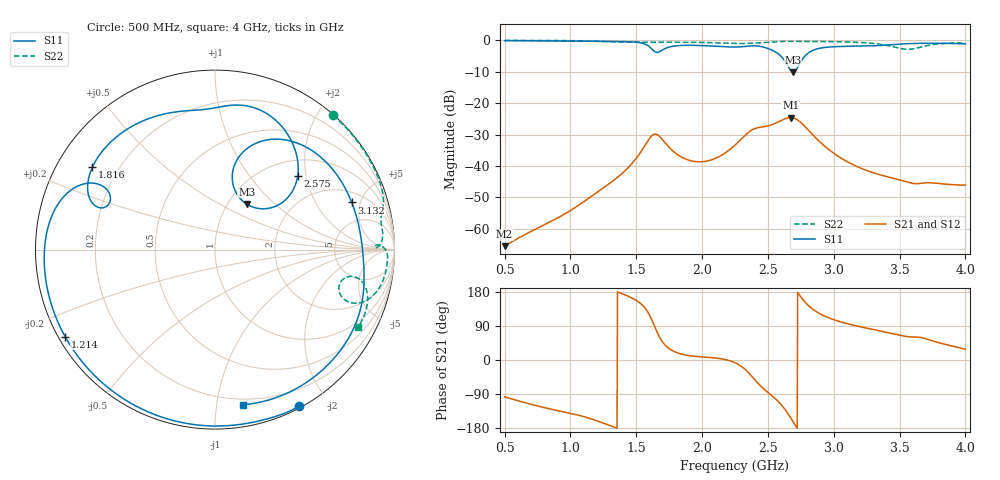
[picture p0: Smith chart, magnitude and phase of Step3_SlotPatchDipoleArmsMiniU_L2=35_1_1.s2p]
! TOUCHSTONE file generated by CST MICROWAVE STUDIO
! Date and time: Tue May 19 00:06:23 2020
! Project name: DualBand_DualMode_Antenna_FD_SteppedDesign.cst
! Parameters = {FPL=20; FPW=20; L=50; ST=10; SW=30; W=52; WF=7; ext=10; gap=1; inset=13}
! Header version: 2015
! Port assignment regex: !\s*Touchstone port\s*([0-9]+)\s*=\s*CST MWS port\s*([0-9]+)\s*\(\"(.*)\"\)(\s*mode\s*([0-9]+))?.*
! Touchstone port assignment:
! Touchstone port 1 = CST MWS port 1 ("")
! Touchstone port 2 = CST MWS port 2 ("")
# GHz S MA R 50
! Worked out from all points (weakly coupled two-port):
!   1006 points, 500 MHz to 4 GHz, reference 50 ohm
!   highest |S21| = -24.57 dB at 2.674 GHz (marker M1); lowest = -65.5 dB at 500 MHz (marker M2)
!   lowest |S11| = -10.2 dB at 2.691 GHz (marker M3), VSWR 1.89, Z = 60.9 + j34.2 ohm
!   |S11| at or under -10 dB: 2.682 GHz to 2.703 GHz (21.03 MHz wide, 0.781 % of centre)
!   |S22| runs from -2.8 to 0.0 dB; largest |S21 - S12| = 4.4e-06
!   S11 on the Smith chart (normalised r, x): 500 MHz: 0.02, -1.67; 1.214 GHz: 0.02, -0.27; 1.816 GHz: 0.11, +0.30; 2.575 GHz: 1.34, +1.79; 3.132 GHz: 2.79, +4.18; 4 GHz: 0.16, -1.19
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0.5  0.9886 -61.7  0.000531 -97.3  0.000531 -97.3  0.9966 48.7
0.7905  0.9817 -97.3  0.001133 -124.8  0.001133 -124.8  0.9958 29.0
1.0845  0.9708 -133.7  0.002556 -147.6  0.002557 -147.6  0.982 17.4
1.214  0.9655 -149.8  0.003971 -162.0  0.003971 -162.0  0.9631 13.8
1.438  0.9504 -179.8  0.009402 168.5  0.009402 168.5  0.9391 10.3
1.578  0.8515 155.9  0.02327 131.6  0.02327 131.6  0.9375 8.4
1.669  0.6499 158.2  0.03063 66.0  0.03063 66.0  0.9377 7.3
1.816  0.8232 146.0  0.01507 18.4  0.01507 18.4  0.938 5.1
2.0295  0.8208 118.5  0.01193 7.5  0.01193 7.5  0.9233 2.0
2.25  0.783 94.5  0.02154 -7.2  0.02154 -7.2  0.8917 0.8
2.4  0.8195 74.1  0.03938 -51.8  0.03938 -51.8  0.9065 1.7
2.5755  0.618 41.8  0.0501 -108.5  0.0501 -108.5  0.9555 -0.7
2.6735  0.3304 44.2  0.05906 -152.9  0.05906 -152.9  0.9627 -3.1
2.691  0.3091 55.2  0.05844 -162.6  0.05844 -162.6  0.9626 -3.5
2.7505  0.4608 77.2  0.04921 166.2  0.04921 166.2  0.9621 -4.7
2.8345  0.6841 63.7  0.0324 135.8  0.0324 135.8  0.9609 -6.4
2.9675  0.784 40.4  0.01796 110.6  0.01795 110.6  0.9553 -9.3
3.132  0.8059 19.0  0.0109 93.3  0.0109 93.3  0.9388 -13.2
3.419  0.8477 -11.6  0.006659 71.8  0.006659 71.8  0.8214 -21.2
3.545  0.883 -26.1  0.005671 62.5  0.005672 62.5  0.7228 -17.3
3.671  0.8975 -41.2  0.005338 58.8  0.00534 58.8  0.7913 -11.0
4  0.8781 -79.7  0.004974 28.5  0.004974 28.5  0.9066 -28.5
